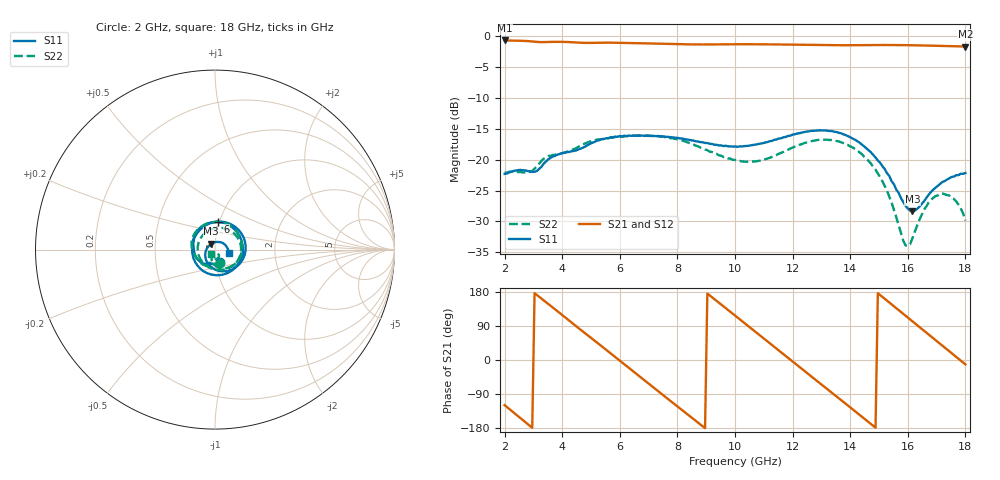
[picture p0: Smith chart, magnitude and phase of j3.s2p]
!Keysight Technologies,P5004A,MY58100454,A.15.10.06
!Date: Monday, July 18, 2022 10:35:06
!Correction: S11(C  2-Port  )
!S21(C  2-Port  )
!S12(C  2-Port  )
!S22(C  2-Port  )
!S2P File: Measurements: S11, S21, S12, S22:
# Hz S  dB  R 50
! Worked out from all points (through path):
!   201 points, 2 GHz to 18 GHz, reference 50 ohm
!   highest |S21| = -0.66 dB at 2 GHz (marker M1); lowest = -1.6 dB at 18 GHz (marker M2)
!   group delay of S21, straight-line fit = 168 ps
!   lowest |S11| = -28.3 dB at 16.16 GHz (marker M3), VSWR 1.08, Z = 47.9 + j3.08 ohm
!   |S11| at or under -10 dB: start of sweep to end of sweep
!   |S22| runs from -34.0 to -16.1 dB; largest |S21 - S12| = 0.00052
!   S11 on the Smith chart (normalised r, x): 2 GHz: 1.05, -0.15; 6 GHz: 0.99, +0.31; 18 GHz: 1.16, -0.05
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2e9  -22.31 -67.9  -0.66 -119.1  -0.66 -119.1  -22.13 -67.8
2.64e9  -21.72 -99.3  -0.72 -159.0  -0.72 -159.0  -22.09 -94.4
3.2e9  -21.50 -115.4  -0.92 166.9  -0.92 166.9  -20.63 -109.3
4e9  -18.93 -157.0  -0.89 118.6  -0.89 118.6  -18.93 -154.1
4.72e9  -18.05 165.4  -1.05 75.1  -1.05 75.0  -17.51 169.4
6e9  -16.17 83.7  -1.03 -1.9  -1.03 -1.9  -16.29 96.5
6.56e9  -16.12 46.2  -1.09 -35.9  -1.09 -35.9  -16.08 65.6
7.36e9  -16.16 -7.3  -1.18 -84.0  -1.18 -84.1  -16.22 21.9
8e9  -16.45 -50.8  -1.25 -122.5  -1.25 -122.6  -16.68 -13.1
8.8e9  -17.14 -103.9  -1.31 -170.3  -1.31 -170.4  -18.05 -57.9
1e10  -17.86 -175.0  -1.28 117.4  -1.27 117.4  -20.05 -131.1
1.072e10  -17.54 146.2  -1.28 73.7  -1.28 73.7  -20.27 174.3
1.152e10  -16.56 103.3  -1.31 25.0  -1.31 25.0  -19.03 111.7
1.208e10  -15.88 73.0  -1.35 -8.9  -1.35 -8.9  -17.87 70.7
1.272e10  -15.31 36.7  -1.40 -47.6  -1.40 -47.7  -16.93 27.6
1.384e10  -16.00 -30.1  -1.43 -115.2  -1.44 -115.2  -17.48 -39.3
1.464e10  -18.46 -80.8  -1.41 -164.0  -1.41 -164.0  -20.24 -82.2
1.536e10  -22.67 -134.8  -1.40 151.7  -1.40 151.7  -26.04 -112.6
1.592e10  -27.47 161.1  -1.42 117.0  -1.42 117.0  -33.89 -92.4
1.616e10  -28.35 122.8  -1.44 102.2  -1.44 102.1  -32.75 -62.2
1.712e10  -23.93 22.3  -1.54 42.8  -1.54 42.8  -25.52 -80.2
1.8e10  -22.15 -15.0  -1.64 -11.5  -1.64 -11.6  -29.86 -135.9
